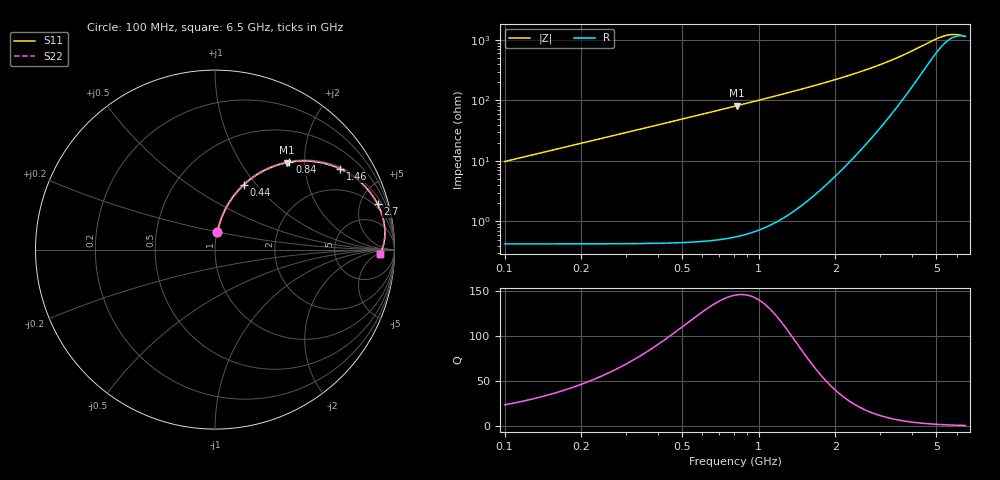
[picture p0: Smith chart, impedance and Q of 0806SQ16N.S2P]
! Coilcraft 0806SQ-16N Air Core Inductor
! 07 March 2008
# MHZ S MA R 50
!Freq  MagS11  AngS11  MagS21  AngS21  MagS12  AngS12  MagS22  AngS22
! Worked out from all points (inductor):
!   321 points, 100 MHz to 6.5 GHz, reference 50 ohm
!   read as one part in series: L = 15.6 nH near 120 MHz
!   highest Q = 146 at 820 MHz (marker M1), where L = 15.9 nH
!   S11 on the Smith chart (normalised r, x): 100 MHz: 1.01, +0.19; 440 MHz: 1.01, +0.86; 840 MHz: 1.02, +1.68; 1.46 GHz: 1.06, +3.07; 2.7 GHz: 1.56, +6.91; 6.5 GHz: 22, -7
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100  0.0967 81.9  0.9911 -5.6  0.9911 -5.6  0.0967 81.9
120  0.1158 81.2  0.9891 -6.7  0.9891 -6.7  0.1158 81.2
160  0.1536 79.6  0.9839 -8.9  0.9839 -8.9  0.1536 79.6
200  0.1908 77.7  0.9775 -11.1  0.9775 -11.1  0.1908 77.7
240  0.2272 75.8  0.9697 -13.2  0.9697 -13.2  0.2272 75.8
340  0.3143 70.8  0.9453 -18.4  0.9453 -18.4  0.3143 70.8
440  0.3945 66.0  0.9149 -23.4  0.9149 -23.4  0.3945 66.0
620  0.5196 58.1  0.8504 -31.5  0.8504 -31.5  0.5197 58.1
820  0.6297 50.3  0.7725 -39.3  0.7725 -39.3  0.6298 50.3
840  0.6392 49.6  0.7647 -40.0  0.7647 -40.0  0.6392 49.6
1000  0.706 44.4  0.7032 -45.2  0.7032 -45.2  0.706 44.4
1180  0.7648 39.3  0.638 -50.2  0.638 -50.2  0.7648 39.3
1460  0.8304 32.8  0.5475 -56.6  0.5475 -56.6  0.8305 32.8
1820  0.8838 26.2  0.4507 -62.6  0.4507 -62.6  0.8839 26.2
2240  0.9198 20.5  0.3613 -67.5  0.3613 -67.5  0.9198 20.5
2700  0.9407 15.7  0.2849 -70.7  0.2849 -70.7  0.9407 15.7
3300  0.952 11.0  0.2094 -71.8  0.2094 -71.8  0.952 11.0
4380  0.9505 5.1  0.1202 -63.8  0.1202 -63.8  0.9505 5.1
4980  0.9438 2.7  0.09145 -51.5  0.09145 -51.5  0.9438 2.7
5440  0.9372 1.2  0.07942 -38.0  0.07942 -38.0  0.9372 1.2
5920  0.9296 -0.2  0.07577 -22.7  0.07577 -22.7  0.9296 -0.2
6500  0.9198 -1.6  0.08052 -7.2  0.08052 -7.2  0.9198 -1.6
